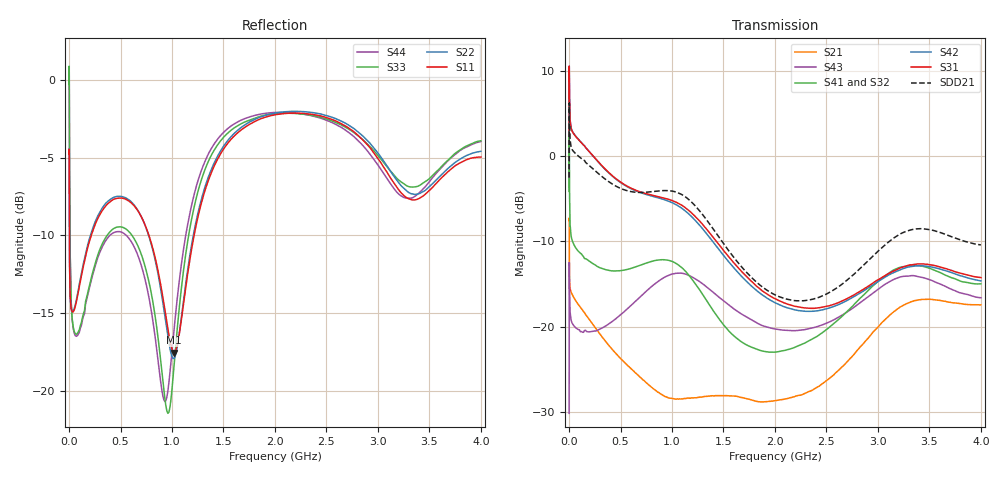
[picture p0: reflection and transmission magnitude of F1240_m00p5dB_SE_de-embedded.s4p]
! Integrated Device Technology
! Corporate Headquarters
! 6024 Silver Creek Valley Road
! San Jose, CA 95138  USA
! Phone:  1-408-284-8200
! Toll Free:  1-800-223-1366
! Webpage:  http://www.idt.com/
! Timing and RF Division
! 515 Groton Road, Suite 102
! Westford, MA 01886-6024
! Device:  F1240
! Description: Dual Intermediate Frequency Digital Variable Gain Amplifier
! Frequency:  10.0 -  500.00 MHz
! Package:  5x5 mm QFN Plastic Package: 32 pin
! Ports:  8 RF, 20 DC
!  Pin  1  = GA3 / Data  Pin 17  = RF OUT_B+
!  Pin  2  = GA4 / CLK  Pin 18  = RF OUT_B-
!  Pin  3  = GA5  Pin 19  = STBY_B
!  Pin  4  = VMODE  Pin 20  = Ground
!  Pin  5  = No Connect  Pin 21  = Ground
!  Pin  6  = GB5  Pin 22  = STB_A
!  Pin  7  = GB4  Pin 23  = RF OUT_A-  = Port 4
!  Pin  8  = GB3  Pin 24  = RF OUT_A+  = Port 3
!  Pin  9  = GB2  Pin 25  = GA0
!  Pin 10  = GB1  Pin 26  = ISET_A
!  Pin 11  = RF IN_B+  Pin 27  = VCC
!  Pin 12  = RF IN_B-  Pin 28  = Ground
!  Pin 13  = Ground  Pin 29  = RF IN_A-  = Port 2
!  Pin 14  = VCC  Pin 30  = RF IN_A+  = Port 1
!  Pin 15  = ISET_B  Pin 31  = GA1
!  Pin 16  = GB0  Pin 32  = GA2 / CSb
! Gain  = +19.5 dB
! State  = 1
! Voltage  = +5.00 V
! Current  = 85.292 mA (one channel only)
! Temperture  =  +25 C
! Test Date  =  2017-10-18
! Board  =  EB4031
! Data:  The device was measured on a custom evaluation board which has
!  individual transmission lines to the RF pins.  Data was collected
!  using a calibrated network analyzer.  The evaluation board was
!  de-embedded using Automatic Fixture Removal.
!  The reference plane is the edge of the package pin.
!  Only Channel A was measured.
!  This data is in single-ended operation.  If your needs are balanced
!  or differential S-parameters then this file needs to be used a
!  linear simulator.
! File Date:  2017-11-10  MJV
! Note:
!  Integrated Device Technology supplies this data as a sample of measured
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# Hz S dB R 100
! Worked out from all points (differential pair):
!   410 points, 500 kHz to 4 GHz, reference 100 ohm
!   strongest paths, dB at 500 kHz, 930 MHz, 1.96 GHz, 2.98 GHz, 4 GHz:
!     S31: 2.7, -4.9, -16.5, -14.7, -14.2
!     S42: 2.7, -5.1, -16.9, -14.9, -14.6
!     S41: -4.1, -12.2, -23.0, -14.9, -15.0
!     S32: -4.1, -12.3, -23.0, -15.3, -15.5
!     S43: -30.2, -14.2, -20.2, -15.8, -16.6
!     S21: -7.5, -28.2, -28.8, -20.3, -17.4
!   taken as a pair (ports 1,2 in; 3,4 out), SDD21 dB: -2.5, -4.0, -16.0, -11.4, -10.4
!   lowest |S11| = -17.6 dB at 1.02 GHz (marker M1), VSWR 1.31, Z = 78 - j8.43 ohm
!   |S11| at or under -10 dB: 3.543 MHz to 216.3 MHz (212.8 MHz wide, 194 % of centre); 775.1 MHz to 1.215 GHz (439.7 MHz wide, 44.2 % of centre)
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500000  -4.76 -5.6  -7.51 -5.8  -30.13 80.7  -36.86 78.7
        -7.52 -5.8  -4.75 -5.6  -36.84 77.5  -30.13 81.8
        2.74 -107.5  -4.10 -109.7  -0.29 0.8  -30.20 -45.0
        -4.13 -108.6  2.73 -106.4  -30.17 -45.2  -0.30 3.1
2000000  -6.33 -37.6  -9.79 -37.7  -20.42 31.8  -28.00 11.2
         -9.80 -37.7  -6.30 -37.6  -27.96 11.0  -20.40 32.1
         10.52 -173.2  3.14 168.0  0.08 -47.6  -12.46 -137.3
         3.10 168.2  10.52 -172.8  -12.45 -137.3  0.04 -47.2
4000000  -10.71 -42.0  -14.08 -30.4  -20.47 10.4  -30.90 -11.8
         -14.08 -30.4  -10.69 -42.3  -30.87 -12.0  -20.47 10.6
         7.49 161.9  -2.96 139.1  -4.37 -81.2  -14.72 176.8
         -3.01 139.3  7.50 162.1  -14.71 176.7  -4.42 -81.1
1.7e8  -11.09 -104.9  -18.73 -54.1  -22.79 -43.8  -35.35 -31.1
       -18.72 -54.1  -10.91 -106.3  -35.43 -30.6  -22.80 -44.1
       0.88 116.6  -12.11 83.5  -14.03 -146.0  -20.61 107.5
       -12.09 83.4  0.89 115.8  -20.57 107.0  -14.18 -145.9
1.02e9  -17.56 -156.4  -28.90 -171.2  -23.22 149.5  -31.26 -168.4
        -28.48 -173.1  -17.94 -153.3  -31.23 -162.8  -23.89 148.6
        -5.30 -93.3  -12.65 167.5  -18.38 -113.1  -14.00 -123.1
        -12.46 163.5  -5.57 -95.9  -13.78 -123.3  -16.07 -107.6
2.86e9  -3.92 97.5  -22.01 -29.0  -25.35 -154.2  -27.60 -137.8
        -21.97 -29.0  -3.65 98.5  -28.41 -125.4  -26.56 -148.9
        -15.62 -67.1  -16.67 -154.1  -3.89 101.9  -17.83 -80.3
        -16.31 -164.8  -15.82 -64.1  -16.90 -78.3  -4.27 95.0
4e9  -4.96 -141.3  -17.48 105.3  -23.83 -40.0  -24.84 -24.1
     -17.44 105.2  -4.59 -139.5  -25.78 -9.0  -25.55 -33.1
     -14.25 42.4  -15.45 -60.7  -3.91 -134.0  -18.12 66.2
     -14.98 -73.9  -14.64 48.4  -16.62 57.6  -3.96 -143.7
